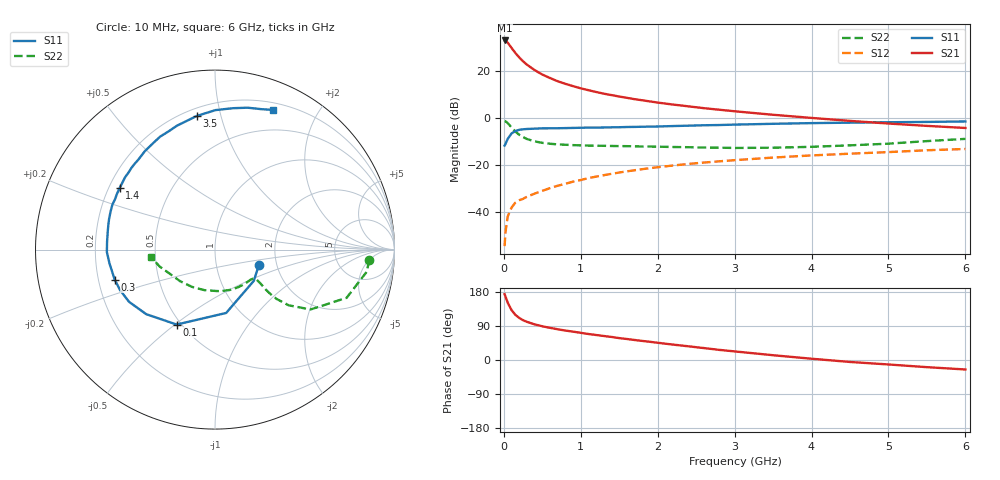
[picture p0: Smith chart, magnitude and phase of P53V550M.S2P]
! SIEMENS Small Signal Semiconductors
! BFP183
! Si NPN RF Bipolar Junction Transistor in SOT143
! VCE = 3.5 V  IC = 50 mA
! Common Emitter S-Parameters:  March  1996
# GHz  S  MA  R  50
!  f  S11  S21  S12  S22
! GHz  MAG  ANG  MAG  ANG  MAG  ANG  MAG  ANG
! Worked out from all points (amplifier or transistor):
!   36 points, 10 MHz to 6 GHz, reference 50 ohm
!   highest |S21| = 32.9 dB at 10 MHz (marker M1)
!   |S21| within 3 dB of that: start of sweep to 96.53 MHz
!   unconditionally stable (mu >= 1): start of sweep to 15.49 MHz; 346.6 MHz to end of sweep
!   at 250 MHz: K = 0.86, MSG = 29.2 dB, |S12| = -34.3 dB
!   at 1.4 GHz: K = 1.36, MAG = 13.2 dB, |S12| = -23.7 dB
!   at 6 GHz: K = 1.05, MAG = 3.1 dB, |S12| = -13.2 dB
!   S11 on the Smith chart (normalised r, x): 10 MHz: 1.61, -0.30; 100 MHz: 0.47, -0.51; 300 MHz: 0.27, -0.14; 1.4 GHz: 0.24, +0.28; 3.5 GHz: 0.25, +0.84; 6 GHz: 0.27, +1.47
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0.01  0.2591 -19.9  44.15 173.8  0.0019 72.1  0.8623 -3.8
0.02  0.2776 -38.8  43.66 168.1  0.0036 77.1  0.8535 -8.4
0.05  0.3584 -80.0  39.71 151.4  0.0081 69.8  0.7811 -20.1
0.1  0.469 -117.1  30.7 131.7  0.0125 56.3  0.628 -32.1
0.15  0.5256 -136.8  23.93 119.1  0.016 50.7  0.5142 -37.1
0.2  0.5604 -148.7  19.24 110.9  0.0179 49.9  0.4388 -38.7
0.25  0.5751 -156.9  15.91 105.0  0.0192 50.5  0.3921 -38.7
0.3  0.5833 -163.4  13.53 100.7  0.0213 52.4  0.3576 -38.1
0.4  0.5927 -172.4  10.37 94.0  0.0248 55.0  0.3185 -36.8
0.5  0.6026 -178.7  8.34 89.0  0.0284 56.4  0.2964 -36.1
0.6  0.6029 175.9  7.046 84.8  0.0324 58.6  0.2834 -35.9
0.7  0.6053 171.2  6.009 81.1  0.0364 60.2  0.2749 -36.1
0.8  0.6095 167.3  5.301 77.7  0.0401 60.4  0.27 -36.8
1.1  0.6243 156.3  3.884 68.6  0.0529 61.1  0.2591 -40.6
1.4  0.6328 147.0  3.057 60.8  0.0652 60.1  0.2542 -45.9
1.7  0.6455 138.2  2.505 52.8  0.0777 58.0  0.2504 -52.4
2.2  0.6734 125.5  1.924 40.6  0.0979 53.7  0.2418 -64.5
2.8  0.7077 111.4  1.496 26.7  0.1201 47.7  0.2339 -81.7
3.5  0.7515 97.7  1.169 12.6  0.1443 41.2  0.2335 -104.5
4.5  0.7943 82.7  0.867 -5.2  0.1745 31.3  0.2623 -137.9
5.5  0.8238 71.8  0.679 -18.9  0.2064 22.6  0.3228 -163.1
6  0.843 67.3  0.613 -25.0  0.2194 17.6  0.3597 -173.6
